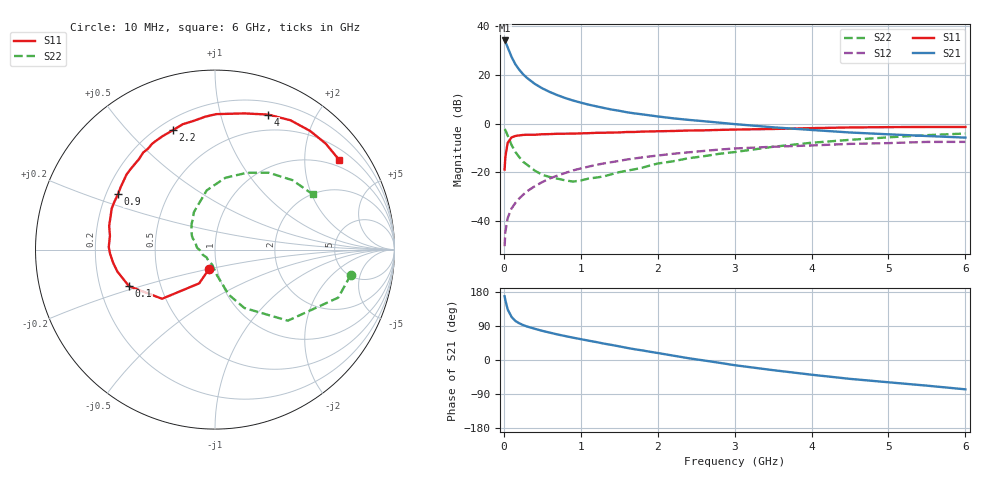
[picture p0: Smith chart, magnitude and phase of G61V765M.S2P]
! SIEMENS Small Signal Semiconductors
! BFG193
! Si NPN RF Bipolar Junction Transistor in SOT223
! VCE = 1.75 V  IC = 65 mA
! Common Emitter S-Parameters:  August  1996
# GHz  S  MA  R  50
!  f  S11  S21  S12  S22
! GHz  MAG  ANG  MAG  ANG  MAG  ANG  MAG  ANG
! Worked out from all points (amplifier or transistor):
!   36 points, 10 MHz to 6 GHz, reference 50 ohm
!   highest |S21| = 34.3 dB at 10 MHz (marker M1)
!   |S21| within 3 dB of that: start of sweep to 51.8 MHz
!   unconditionally stable (mu >= 1): start of sweep to 13.99 MHz; 219.1 MHz to 2.911 GHz; 3.191 GHz to 3.638 GHz
!   at 250 MHz: K = 1.03, MAG = 23.8 dB, |S12| = -29.3 dB
!   at 1.4 GHz: K = 1.11, MAG = 8.9 dB, |S12| = -15.9 dB
!   at 6 GHz: K = 0.99, MSG = 0.9 dB, |S12| = -7.5 dB
!   S11 on the Smith chart (normalised r, x): 10 MHz: 0.91, -0.20; 100 MHz: 0.33, -0.18; 900 MHz: 0.25, +0.25; 2.2 GHz: 0.26, +0.68; 4 GHz: 0.33, +1.42; 6 GHz: 0.78, +2.89
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0.01  0.1136 -107.2  51.59 168.1  0.003 79.0  0.77 -10.5
0.02  0.2076 -115.1  48.48 157.8  0.0059 72.9  0.7366 -21.3
0.05  0.4024 -137.1  37.12 133.4  0.0114 64.0  0.5671 -44.3
0.1  0.5211 -157.0  23.71 113.8  0.0179 62.6  0.364 -63.3
0.15  0.5574 -167.3  16.67 103.0  0.0233 64.5  0.2614 -73.2
0.2  0.5729 -172.8  12.9 97.0  0.0288 66.2  0.2048 -77.1
0.25  0.5848 -177.7  10.42 92.2  0.0342 67.3  0.1644 -82.0
0.3  0.592 178.6  8.758 88.5  0.0403 68.6  0.1433 -85.6
0.4  0.5904 172.5  6.624 82.5  0.0512 68.4  0.1084 -92.6
0.5  0.6047 167.2  5.33 76.9  0.0627 67.3  0.0882 -99.0
0.6  0.6092 163.1  4.463 72.1  0.0744 66.1  0.0795 -106.4
0.7  0.6193 158.4  3.84 67.3  0.0857 64.7  0.0734 -116.4
0.9  0.6224 150.2  2.994 58.9  0.1089 60.9  0.0641 -137.7
1.1  0.6366 143.3  2.465 51.1  0.1302 57.0  0.0738 -156.7
1.6  0.6728 126.5  1.714 32.0  0.1826 45.5  0.1075 167.3
2.2  0.7054 109.5  1.287 11.6  0.2396 31.0  0.1679 141.3
3  0.7548 89.5  0.978 -13.7  0.3077 11.8  0.2599 112.5
3.5  0.7761 77.9  0.841 -26.8  0.3344 -1.5  0.3335 97.9
4  0.8085 68.5  0.741 -38.8  0.3556 -11.3  0.4042 81.8
4.5  0.8344 59.7  0.657 -49.8  0.3828 -21.6  0.4637 67.4
5.5  0.8539 43.8  0.556 -67.7  0.4202 -44.8  0.5795 41.9
6  0.8535 36.0  0.515 -77.4  0.4206 -57.9  0.6255 29.5
